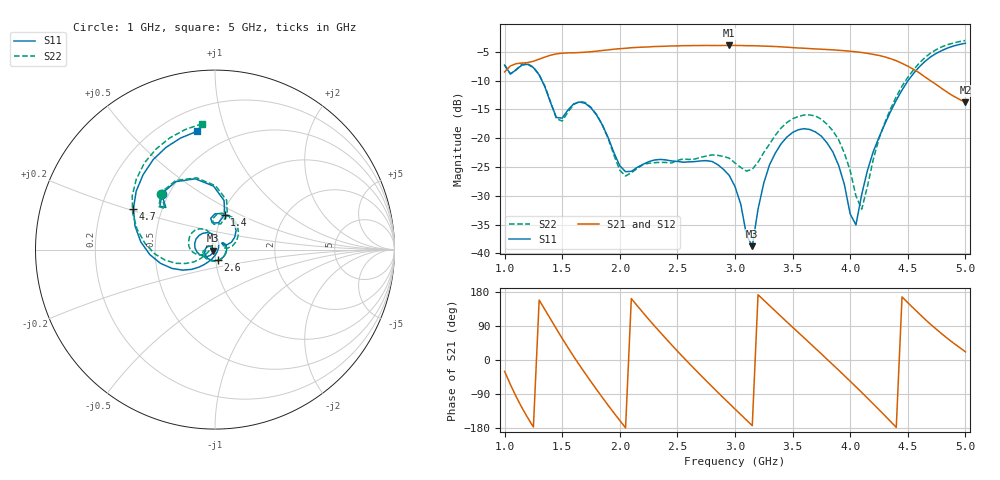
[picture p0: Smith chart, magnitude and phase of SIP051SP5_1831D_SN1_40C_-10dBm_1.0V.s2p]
# GHz  S  dB  R  50
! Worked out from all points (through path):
!   81 points, 1 GHz to 5 GHz, reference 50 ohm
!   highest |S21| = -3.91 dB at 2.95 GHz (marker M1); lowest = -13.8 dB at 5 GHz (marker M2)
!   lowest |S11| = -38.7 dB at 3.15 GHz (marker M3), VSWR 1.02, Z = 49 - j0.552 ohm
!   |S11| at or under -10 dB: 1.323 GHz to 4.503 GHz (3.179 GHz wide, 109 % of centre)
!   |S22| runs from -32.3 to -3.0 dB; largest |S21 - S12| = 0.0026
!   S11 on the Smith chart (normalised r, x): 1 GHz: 0.46, +0.35; 1.4 GHz: 1.03, +0.42; 2.6 GHz: 1.03, -0.12; 4.7 GHz: 0.34, +0.21; 5 GHz: 0.34, +0.80
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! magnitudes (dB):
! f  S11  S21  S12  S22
! 1 GHz  -7.3  -8.5  -8.5  -7.3
! 1.25 GHz  -7.8  -6.7  -6.6  -7.7
! 1.4 GHz  -13.9  -5.6  -5.6  -13.8
! 1.5 GHz  -16.5  -5.3  -5.2  -17.0
! 1.7 GHz  -14.0  -5.1  -5.1  -13.8
! 2.05 GHz  -25.8  -4.4  -4.4  -26.6
! 2.35 GHz  -23.7  -4.1  -4.1  -24.2
! 2.6 GHz  -24.1  -3.9  -3.9  -23.7
! 2.95 GHz  -26.5  -3.9  -3.9  -23.5
! 3 GHz  -28.4  -3.9  -3.9  -24.3
! 3.15 GHz  -38.7  -4.0  -4.0  -25.4
! 3.25 GHz  -27.8  -4.0  -4.0  -22.5
! 3.35 GHz  -22.6  -4.1  -4.1  -19.5
! 3.5 GHz  -19.0  -4.3  -4.3  -16.6
! 3.7 GHz  -18.9  -4.5  -4.5  -16.2
! 3.9 GHz  -24.7  -4.8  -4.7  -20.3
! 4.05 GHz  -35.1  -5.0  -5.0  -30.1
! 4.1 GHz  -29.8  -5.1  -5.1  -32.3
! 4.25 GHz  -19.9  -5.6  -5.7  -20.1
! 4.35 GHz  -15.4  -6.2  -6.2  -14.9
! 4.7 GHz  -5.9  -10.1  -10.0  -5.2
! 5 GHz  -3.5  -13.8  -13.8  -3.0
